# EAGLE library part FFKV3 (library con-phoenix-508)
PHOENIX
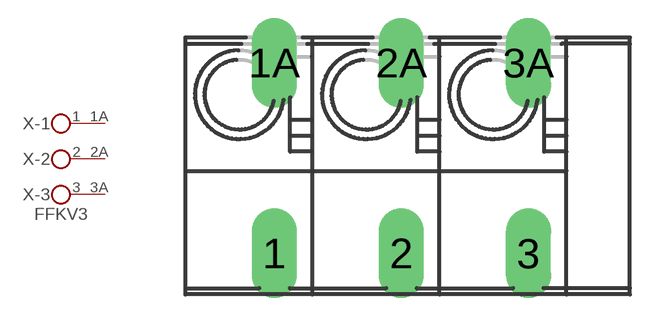
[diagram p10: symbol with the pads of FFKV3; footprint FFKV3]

Designator prefix X; gates -1=KL2 -2=KL2 -3=KL2V

## FFKV3 (OC_FARNELL: unknown; OC_NEWARK: unknown)  [FFKV3]
1  -1:1  pas
1A  -1:2  pas
2  -2:1  pas
2A  -2:2  pas
3  -3:1  pas
3A  -3:2  pas

## Footprint FFKV3 (pad centres in mm)
PHOENIX
drill 1.194 long: 1 -5.08,-3.81; 1A -5.08,3.81; 2 0,-3.81; 2A 0,3.81; 3 5.08,-3.81; 3A 5.08,3.81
